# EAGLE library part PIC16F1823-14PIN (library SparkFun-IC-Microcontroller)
MCU PIC FLASH 14TSSOP Datasheet SparkFun Products ZX Distance and Gesture Sensor (SEN-12780) Short timer
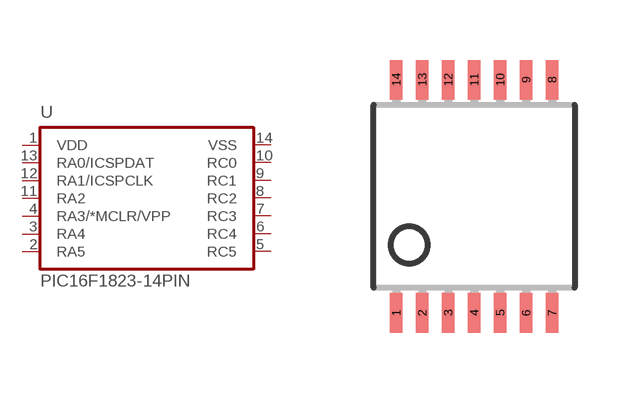
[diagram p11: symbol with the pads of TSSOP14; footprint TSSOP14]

Designator prefix -

## PIC16F1823-14PINTSSOP (PROD_ID: IC-11992)  [TSSOP14]
1  VDD  pwr
2  RA5
3  RA4
4  RA3/*MCLR/VPP  in
5  RC5
6  RC4
7  RC3
8  RC2
9  RC1
10  RC0
11  RA2
12  RA1/ICSPCLK
13  RA0/ICSPDAT
14  VSS  pwr

## Footprint TSSOP14 (pad centres in mm)
Thin Shrink Small Outline Plastic 14
smd 0.305 x 0.991: 1 -1.95,-2.918; 2 -1.3,-2.918; 3 -0.65,-2.918; 4 0,-2.918; 5 0.65,-2.918; 6 1.3,-2.918; 7 1.95,-2.918; 8 1.95,2.918; 9 1.3,2.918; 10 0.65,2.918; 11 0,2.918; 12 -0.65,2.918; 13 -1.3,2.918; 14 -1.95,2.918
